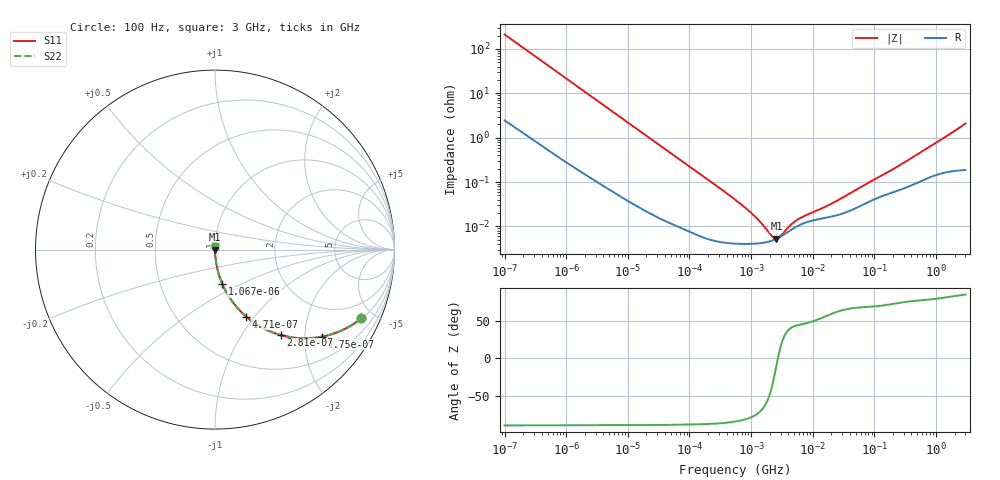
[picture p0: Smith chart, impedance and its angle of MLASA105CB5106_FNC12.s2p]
! MLASA105CB5106_FNC12  S-PARAMETER MODEL  ( Standard Model )
! Model Generated by TAIYO YUDEN Corporation (http://www.ty-top.com)
! Version 1.0
! TAIYO YUDEN Control No. 241206
! Copyright(c) 2024 TAIYO YUDEN CO.,LTD. All Rights Reserved.
! Product Description (link to TY-COMPAS)
! https://ds.yuden.co.jp/TYCOMPAS/or/detail?pn=MLASA105CB5106MFNC12&u=M
! Products Name : Multilayer Ceramic Capacitors
! Characteristics :
!  Capacitance : 10 [uF] , Rated Voltage : 4 [V] , TCC : X5R
!  Case Size : 1.0 x 0.5 / 0.039 x 0.02 [mm/inch] , Thickness : 0.5 / 0.02 [mm/inch]
!  (Conditions: Temperature = 25 [degC] , DC Bias Voltage = 0 [V])
! External Node Assignments :
!  1  o---| |---o  2
! GND o---------o GND
! Frequency Range : 100Hz  -  3GHz  [ 401 STEP ]
# MHZ S RI R 50
! Freq[MHz].  S11 Real  S11 Imag  S21 Real  S21 Imag  S12 Real  S12 Imag  S22 Real  S22 Imag
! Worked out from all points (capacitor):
!   401 points, 100 Hz to 3 GHz, reference 50 ohm
!   read as one part in series: C = 7.5 uF near 109 Hz
!   lowest |Z| = 5.32 mohm at 2.579 MHz (marker M1)
!   series resonance near 2.72 MHz, so ESL is about 460 pH
!   S11 on the Smith chart (normalised r, x): 100 Hz: 1.05, -4.24; 175 Hz: 1.03, -2.43; 281 Hz: 1.02, -1.52; 471 Hz: 1.01, -0.91; 1.067 kHz: 1.01, -0.40; 3 GHz: 1.00, +0.04
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0.0001  0.815 -0.3826  0.185 0.3826  0.185 0.3826  0.815 -0.3826
0.000119  0.7588 -0.422  0.2412 0.422  0.2412 0.422  0.7588 -0.422
0.000175  0.5956 -0.4849  0.4044 0.4849  0.4044 0.4849  0.5956 -0.4849
0.000227  0.4702 -0.4932  0.5298 0.4932  0.5298 0.4932  0.4702 -0.4932
0.000281  0.3679 -0.4762  0.6321 0.4762  0.6321 0.4762  0.3679 -0.4762
0.000471  0.1748 -0.3737  0.8252 0.3737  0.8252 0.3737  0.1748 -0.3737
0.000664  0.0978 -0.2908  0.9022 0.2908  0.9022 0.2908  0.0978 -0.2908
0.001067  0.0416 -0.1934  0.9584 0.1934  0.9584 0.1934  0.0416 -0.1934
0.001788  0.0161 -0.1191  0.9839 0.1191  0.9839 0.1191  0.0161 -0.1191
0.005476  0.00221 -0.0399  0.9978 0.0399  0.9978 0.0399  0.00221 -0.0399
0.031977  0.000203 -0.00696  0.9998 0.00696  0.9998 0.00696  0.000203 -0.00696
0.547723  4.11e-05 -0.000401  1 0.000401  1 0.000401  4.11e-05 -0.000401
0.958445  4.04e-05 -0.000209  1 0.000209  1 0.000209  4.04e-05 -0.000209
1.6065  4.3e-05 -9.25e-05  1 9.25e-05  1 9.25e-05  4.3e-05 -9.25e-05
1.75092  4.39e-05 -7.61e-05  1 7.61e-05  1 7.61e-05  4.39e-05 -7.61e-05
2.579298  5.25e-05 -8.59e-06  0.9999 8.59e-06  0.9999 8.59e-06  5.25e-05 -8.59e-06
4.141163  7.81e-05 6.22e-05  0.9999 -6.22e-05  0.9999 -6.22e-05  7.81e-05 6.22e-05
6.10039  0.000107 0.000106  0.9999 -0.000106  0.9999 -0.000106  0.000107 0.000106
9.794414  0.000135 0.000155  0.9999 -0.000155  0.9999 -0.000155  0.000135 0.000155
22.1892  0.000172 0.000303  0.9998 -0.000303  0.9998 -0.000303  0.000172 0.000303
175.1444  0.000553 0.00165  0.9994 -0.00165  0.9994 -0.00165  0.000553 0.00165
3000  0.00229 0.0206  0.9977 -0.0206  0.9977 -0.0206  0.00229 0.0206
